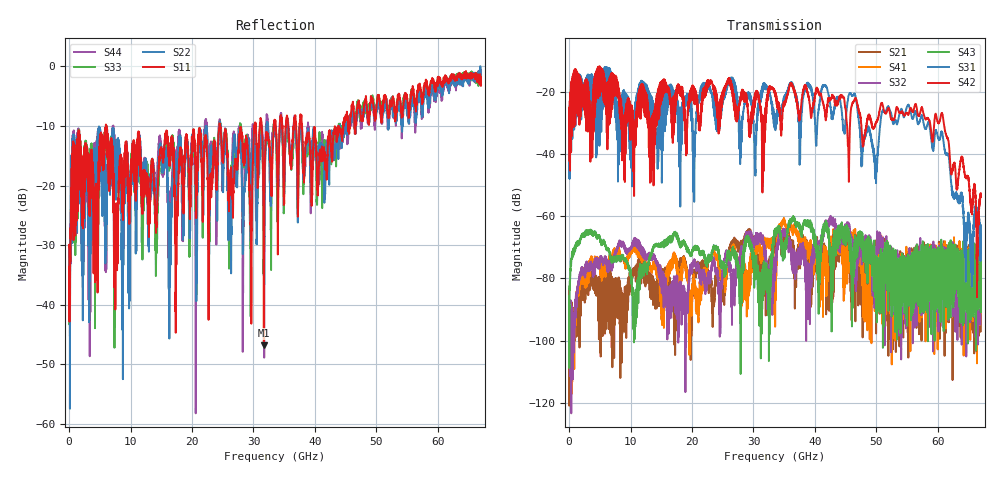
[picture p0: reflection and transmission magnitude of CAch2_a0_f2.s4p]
!Agilent Technologies,N5247A,US51170199,A.09.90.13
!Agilent N5247A: A.09.90.13
!Date: Thursday, October 18, 2018 09:50:29
!Correction: S11(Full 4 Port(1,2,3,4))
!S12(Full 4 Port(1,2,3,4))
!S13(Full 4 Port(1,2,3,4))
!S14(Full 4 Port(1,2,3,4))
!S21(Full 4 Port(1,2,3,4))
!S22(Full 4 Port(1,2,3,4))
!S23(Full 4 Port(1,2,3,4))
!S24(Full 4 Port(1,2,3,4))
!S31(Full 4 Port(1,2,3,4))
!S32(Full 4 Port(1,2,3,4))
!S33(Full 4 Port(1,2,3,4))
!S34(Full 4 Port(1,2,3,4))
!S41(Full 4 Port(1,2,3,4))
!S42(Full 4 Port(1,2,3,4))
!S43(Full 4 Port(1,2,3,4))
!S44(Full 4 Port(1,2,3,4))
!S4P File: Measurements: <S11,S12,S13,S14>,
!<S21,S22,S23,S24>,
!<S31,S32,S33,S34>,
!<S41,S42,S43,S44>:
# Hz S  dB  R 50
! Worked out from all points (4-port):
!   6701 points, 10 MHz to 67 GHz, reference 50 ohm
!   strongest paths, dB at 10 MHz, 16.76 GHz, 33.51 GHz, 50.25 GHz, 67 GHz:
!     S42: -33.0, -27.6, -20.9, -28.5, -52.8
!     S31: -33.4, -21.5, -28.5, -38.7, -62.9
!     S43: -85.7, -66.6, -64.3, -90.1, -73.8
!     S32: -86.3, -81.1, -80.7, -68.7, -72.2
!     S41: -85.5, -74.7, -82.1, -78.2, -73.2
!     S21: -83.1, -84.3, -67.5, -78.8, -73.4
!   lowest |S11| = -46.8 dB at 31.69 GHz (marker M1), VSWR 1.01, Z = 49.9 + j0.432 ohm
!   |S11| at or under -10 dB: start of sweep to 5.983 GHz; 6.1 GHz to 24.46 GHz (18.36 GHz wide, 120 % of centre); 37.91 GHz to 43.82 GHz (5.915 GHz wide, 14.5 % of centre)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
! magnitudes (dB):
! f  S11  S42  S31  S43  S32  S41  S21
! 10 MHz  -30.3  -33.0  -33.4  -85.7  -86.3  -85.5  -83.1
! 5.989 GHz  -9.9  -18.3  -12.2  -70.1  -73.5  -75.3  -77.7
! 31.69 GHz  -46.8  -29.6  -18.4  -74.5  -69.6  -68.5  -79.7
! 46.31 GHz  -7.7  -23.3  -20.9  -69.9  -70.2  -64.5  -76.6
! 49.89 GHz  -8.5  -30.1  -44.0  -83.9  -73.6  -77.6  -72.6
! 55.21 GHz  -7.3  -27.4  -24.2  -86.4  -77.2  -81.1  -71.5
! 67 GHz  -3.2  -52.8  -62.9  -73.8  -72.2  -73.2  -73.4
